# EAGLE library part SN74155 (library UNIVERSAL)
RS232 DRIVER - RECEIVER
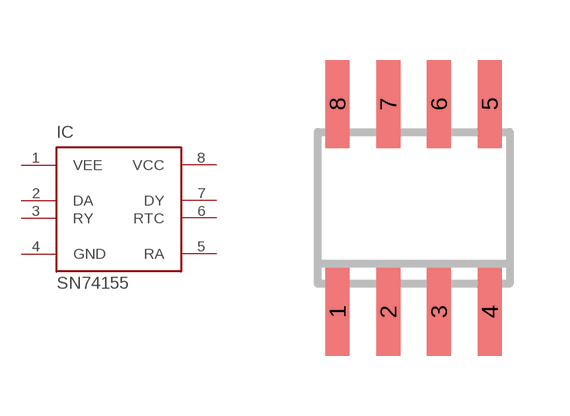
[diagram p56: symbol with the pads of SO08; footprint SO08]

Designator prefix IC

## SN74155  [SO08]
1  VEE  pwr
2  DA  in
3  RY  out
4  GND  pwr
5  RA  in
6  RTC  in
7  DY  out
8  VCC  pwr

## Footprint SO08 (pad centres in mm)
smd 0.6 x 2.2: 1 0,-0.06; 2 1.27,-0.06; 3 2.54,-0.06; 4 3.81,-0.06; 5 3.81,5.14; 6 2.54,5.14; 7 1.27,5.14; 8 0,5.14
